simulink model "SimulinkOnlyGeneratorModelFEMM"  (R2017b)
settings: Solver=ode1  StartTime=0.0  StopTime=0.02  FixedStep=1e-4  RelTol=1e-3

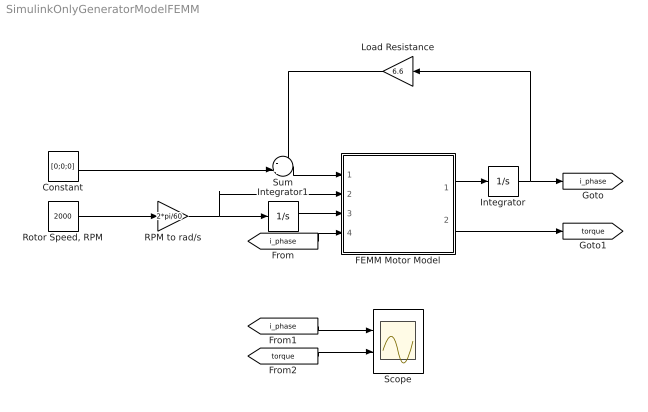
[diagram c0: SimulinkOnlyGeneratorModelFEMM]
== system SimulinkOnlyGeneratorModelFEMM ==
  Constant : Constant  Value=[0;0;0]
  FEMM Motor Model : Subsystem
  Integrator : Integrator
  Integrator1 : Integrator
  Load Resistance : Gain  Gain=6.6
  RPM to rad/s : Gain  Gain=2*pi/60
  "Rotor Speed, RPM" : Constant  Value=2000
  Scope : Scope  NumInputPorts=2
  Sum : Sum  Inputs=-+|
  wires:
  Integrator1/1 -> FEMM Motor Model/3(tta)
  FEMM Motor Model/1(dxdt) -> Integrator/1
  RPM to rad/s/1 -> FEMM Motor Model/2(omega), Integrator1/1
  "Rotor Speed, RPM"/1 -> RPM to rad/s/1
  [i_phase] -> FEMM Motor Model/4(x)
  Integrator/1 -> Load Resistance/1, [i_phase]
  FEMM Motor Model/2(tq) -> [torque]
  [i_phase] -> Scope/1
  [torque] -> Scope/2
  Sum/1 -> FEMM Motor Model/1(u)
  Load Resistance/1 -> Sum/1
  Constant/1 -> Sum/2

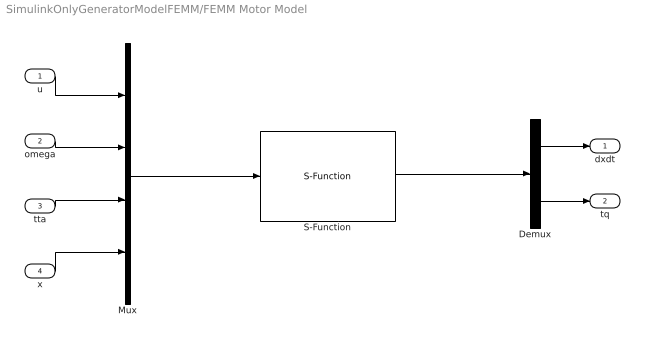
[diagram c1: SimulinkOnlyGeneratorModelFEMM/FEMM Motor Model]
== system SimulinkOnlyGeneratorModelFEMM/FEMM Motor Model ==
  u : Inport
  omega : Inport  Port=2
  tta : Inport  Port=3
  x : Inport  Port=4
  Demux : Demux  Outputs=[3 1]
  Mux : Mux  Inputs=[3 1 1 3]
  S-Function : S-Function  FunctionName=MotorModelFEMM  SFunctionDeploymentMode=off  EnableBusSupport=off
  dxdt : Outport
  tq : Outport  Port=2
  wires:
  u/1 -> Mux/1
  omega/1 -> Mux/2
  tta/1 -> Mux/3
  x/1 -> Mux/4
  Demux/1 -> dxdt/1
  Demux/2 -> tq/1
  S-Function/1 -> Demux/1
  Mux/1 -> S-Function/1
